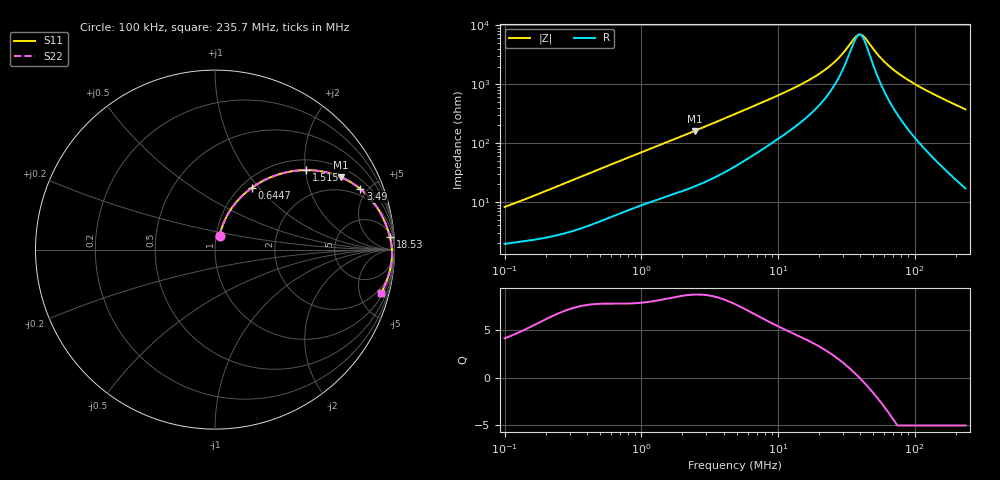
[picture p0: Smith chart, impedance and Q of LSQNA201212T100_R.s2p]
! LSQNA201212T100_R  S-PARAMETER MODEL  ( General Type )
! Model Generated by TAIYO YUDEN Corporation (http://www.ty-top.com)
! Version 2.0
! TAIYO YUDEN Control No. 100810NF25SB-FKC
! Copyright(c) 2007 TAIYO YUDEN CO.,LTD. All Rights Reserved.
! Product Description (link to TY-COMPAS)
! https://ds.yuden.co.jp/TYCOMPAS/or/detail?pn=LSQNA201212T100KR&u=M
! Products Name : Inductors
! Characteristics :
!  Inductance : 10 uH , SRF(min) : 32 MHz , DC Resistance(max) : 0.65 Ohm
!  Rated Current : Saturation :200 mA , Temp Rise : 520 mA (40 degC)
!  Case Size : 2.0 x 1.25 / 0.079 x 0.049 [mm/inch] , Thickness : 1.25 / 0.049 [mm/inch]
!  (Conditions: Temperature = 25 degC , DC Bias Current/Voltage = 0A / 0V)
! External Node Assignments :
!  1  o---GGG---o  2
! GND o---------o GND
! Frequency Range : 0.1MHz  -  235.669543MHz  [ 402 STEP ]
# MHz S RI R 50
! Freq[MHz].  S11 Real  S11 Imag  S21 Real  S21 Imag  S12 Real  S12 Imag  S22 Real  S22 Imag
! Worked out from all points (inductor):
!   401 points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, 100 kHz to 235.7 MHz, reference 50 ohm
!   read as one part in series: L = 12.4 uH near 104 kHz
!   highest Q = 8.7 at 2.461 MHz (marker M1), where L = 10.4 uH
!   self-resonance near 39.51 MHz
!   S11 on the Smith chart (normalised r, x): 100 kHz: 1.04, +0.16; 644.7 kHz: 1.12, +0.92; 1.515 MHz: 1.25, +2.02; 3.49 MHz: 1.53, +4.49; 18.53 MHz: 8, +26; 235.7 MHz: 1.34, -7.50
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0.1  0.0251 0.0766  0.9749 -0.0766  0.9749 -0.0766  0.0251 0.0766
0.193484  0.0436 0.1374  0.9564 -0.1374  0.9564 -0.1374  0.0436 0.1374
0.367165  0.0967 0.2364  0.9033 -0.2364  0.9033 -0.2364  0.0967 0.2364
0.644693  0.2057 0.3448  0.7943 -0.3448  0.7943 -0.3448  0.2057 0.3448
1.348099  0.4601 0.4406  0.5399 -0.4406  0.5399 -0.4406  0.4601 0.4406
1.514629  0.5082 0.443  0.4918 -0.443  0.4918 -0.443  0.5082 0.443
2.460794  0.7016 0.4037  0.2984 -0.4037  0.2984 -0.4037  0.7016 0.4037
3.490027  0.8095 0.3381  0.1905 -0.3381  0.1905 -0.3381  0.8095 0.3381
4.854581  0.8786 0.268  0.1214 -0.268  0.1214 -0.268  0.8786 0.268
10.76001  0.9554 0.1312  0.0446 -0.1312  0.0446 -0.1312  0.9554 0.1312
17.8243  0.9742 0.0728  0.0258 -0.0728  0.0258 -0.0728  0.9742 0.0728
18.52994  0.9752 0.0689  0.0248 -0.0689  0.0248 -0.0689  0.9752 0.0689
26.28014  0.9821 0.0359  0.0179 -0.0359  0.0179 -0.0359  0.9821 0.0359
30.10531  0.9838 0.0238  0.0162 -0.0238  0.0162 -0.0238  0.9838 0.0238
36.55532  0.9855 0.0068  0.0145 -0.0068  0.0145 -0.0068  0.9855 0.0068
39.50697  0.9859 1.2e-05  0.0141 -1.2e-05  0.0141 -1.2e-05  0.9859 1.2e-05
42.69694  0.9862 -0.00682  0.0138 0.00682  0.0138 0.00682  0.9862 -0.00682
53.89715  0.9862 -0.0279  0.0138 0.0279  0.0138 0.0279  0.9862 -0.0279
65.44454  0.9853 -0.0467  0.0147 0.0467  0.0147 0.0467  0.9853 -0.0467
82.61188  0.9826 -0.0716  0.0174 0.0716  0.0174 0.0716  0.9826 -0.0716
108.4109  0.9767 -0.1052  0.0233 0.1052  0.0233 0.1052  0.9767 -0.1052
235.6695  0.9242 -0.243  0.0758 0.243  0.0758 0.243  0.9242 -0.243
